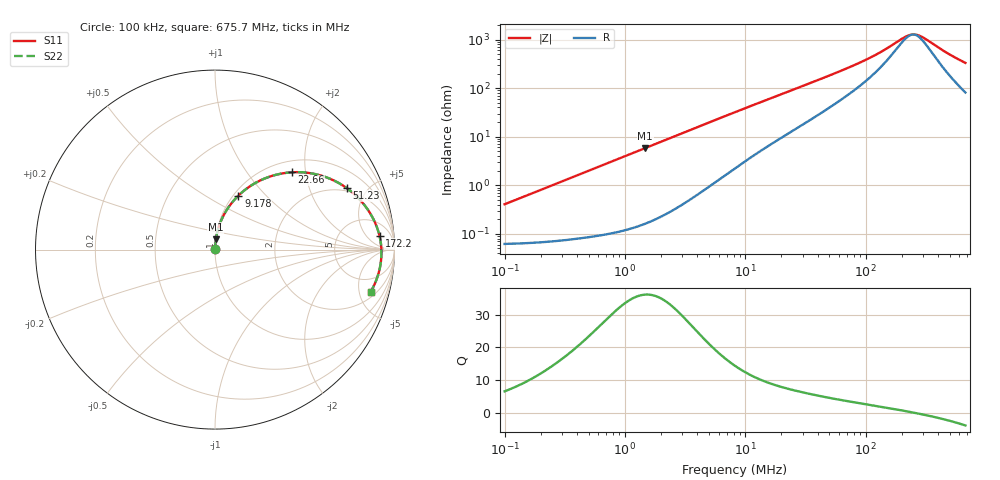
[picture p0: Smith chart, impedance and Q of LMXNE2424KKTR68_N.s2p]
! LMXNE2424KKTR68_N  S-PARAMETER MODEL  ( General Type )
! Model Generated by TAIYO YUDEN Corporation (https://www.yuden.co.jp/en/)
! Version 1.0
! TAIYO YUDEN Control No. 191023NI43SB-FBB
! Copyright(c) 2019 TAIYO YUDEN CO.,LTD. All Rights Reserved.
! Product Description (link to TY-COMPAS)
! https://ds.yuden.co.jp/TYCOMPAS/or/detail?pn=LMXNE2424KKTR68NN&u=M
! Products Name : Inductors
! Characteristics :
!  Inductance : 0.68 uH , SRF(min) : 120 MHz , DC Resistance(max) : 0.072 Ohm
!  Rated Current : Saturation :2200 mA , Temp Rise : 1570 mA (40 degC)
!  Case Size : 2.4 x 2.4 / 0.095 x 0.095 [mm/inch] , Thickness : 1 / 0.039 [mm/inch]
!  (Conditions: Temperature = 25 degC , DC Bias Current/Voltage = 0A / 0V)
! External Node Assignments :
!  1  o---GGG---o  2
! GND o---------o GND
! Frequency Range : 0.1MHz  -  675.68652MHz  [ 402 STEP ]
# MHz S RI R 50
! Freq[MHz].  S11 Real  S11 Imag  S21 Real  S21 Imag  S12 Real  S12 Imag  S22 Real  S22 Imag
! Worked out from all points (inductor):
!   401 points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, 100 kHz to 675.7 MHz, reference 50 ohm
!   read as one part in series: L = 639 nH near 104.5 kHz
!   highest Q = 36.1 at 1.473 MHz (marker M1), where L = 629 nH
!   self-resonance near 247.7 MHz
!   S11 on the Smith chart (normalised r, x): 100 kHz: 1.00, +0.01; 9.178 MHz: 1.05, +0.71; 22.66 MHz: 1.23, +1.68; 51.23 MHz: 1.83, +3.64; 172.2 MHz: 12, +12; 675.7 MHz: 2.62, -6.42
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0.1  0.000636 0.00401  0.9994 -0.00401  0.9994 -0.00401  0.000636 0.00401
0.438008  0.00112 0.0174  0.9989 -0.0174  0.9989 -0.0174  0.00112 0.0174
1.472558  0.00497 0.0579  0.995 -0.0579  0.995 -0.0579  0.00497 0.0579
1.918513  0.00782 0.0751  0.9922 -0.0751  0.9922 -0.0751  0.00782 0.0751
4.532782  0.0379 0.1701  0.9621 -0.1701  0.9621 -0.1701  0.0379 0.1701
8.403244  0.1129 0.2829  0.8871 -0.2829  0.8871 -0.2829  0.1129 0.2829
9.177924  0.1304 0.3009  0.8696 -0.3009  0.8696 -0.3009  0.1304 0.3009
13.95267  0.2432 0.3809  0.7568 -0.3809  0.7568 -0.3809  0.2432 0.3809
22.66174  0.4273 0.4306  0.5727 -0.4306  0.5727 -0.4306  0.4273 0.4306
36.00435  0.6154 0.4045  0.3846 -0.4045  0.3846 -0.4045  0.6154 0.4045
51.23241  0.7335 0.343  0.2665 -0.343  0.2665 -0.343  0.7335 0.343
69.75669  0.8095 0.2755  0.1905 -0.2755  0.1905 -0.2755  0.8095 0.2755
97.09599  0.8655 0.2006  0.1345 -0.2006  0.1345 -0.2006  0.8655 0.2006
123.7426  0.8932 0.147  0.1068 -0.147  0.1068 -0.147  0.8932 0.147
157.702  0.9119 0.0949  0.0881 -0.0949  0.0881 -0.0949  0.9119 0.0949
172.2403  0.9168 0.0762  0.0832 -0.0762  0.0832 -0.0762  0.9168 0.0762
224.4022  0.9258 0.0208  0.0742 -0.0208  0.0742 -0.0208  0.9258 0.0208
245.0894  0.9271 0.00225  0.0729 -0.00225  0.0729 -0.00225  0.9271 0.00225
267.6837  0.9275 -0.0164  0.0725 0.0164  0.0725 0.0164  0.9275 -0.0164
305.5401  0.9266 -0.0448  0.0734 0.0448  0.0734 0.0448  0.9266 -0.0448
507.316  0.9016 -0.162  0.0984 0.162  0.0984 0.162  0.9016 -0.162
675.6865  0.8668 -0.2362  0.1332 0.2362  0.1332 0.2362  0.8668 -0.2362
